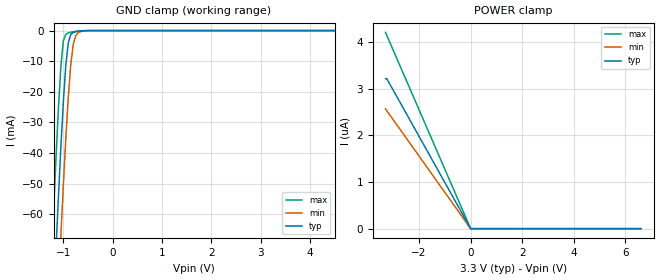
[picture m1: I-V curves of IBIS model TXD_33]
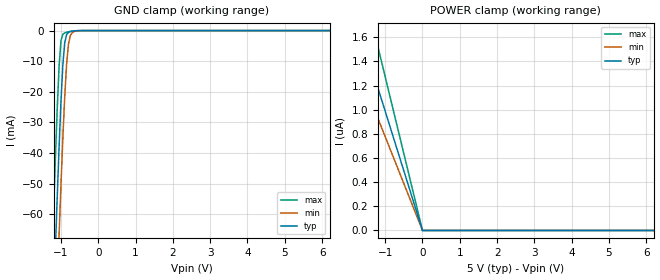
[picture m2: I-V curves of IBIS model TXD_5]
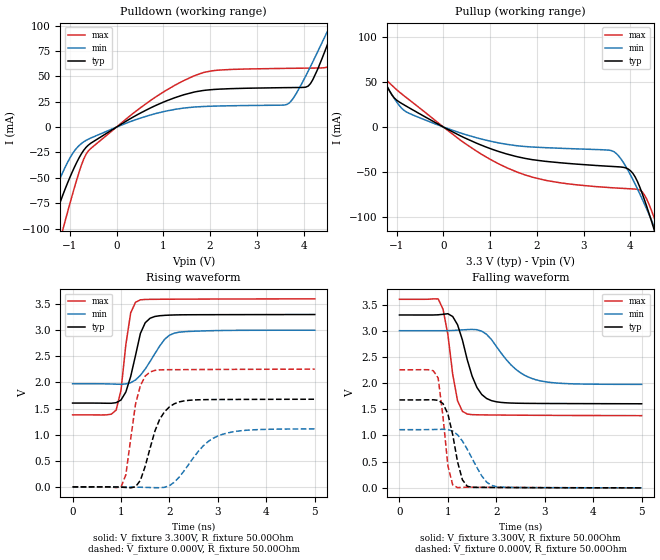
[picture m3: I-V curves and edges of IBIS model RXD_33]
| Texas Instruments Incorporated
| Isolated CAN Transceiver
| Marketing part#   Voltage Range   Package-type   #pins/pkg drawing
| ISO1050DUBR   3V - 5.5V   SOP   8-pin DUB
[IBIS Ver]   4.0
[File name]   iso1050.ibs
[File Rev]   1.0
[Date]   09/04/2009
[Source]   Model built from TISPICED simulations at:
   Texas Instruments Incorporated.
   Analog-eLab, HPA
   12500 TI Blvd
   Dallas, TX -75243
   For Support e-mail: elab_ibis@list.ti.com
[Notes]   Revision History
   Rev 1.0: 09/04/2009
   - Initial model not matched to silicon
   - ccomp values are based on PVT settings:
   MIN: Low Voltage, High Temperature, Weak Process
   TYP: Nominal Voltage, Nominal Temperature, Nominal Process
   MAX: High Voltage, Low Temperature, Fast Process
   - User may change ccomp in the order of number values as
   per end simulator used
[Disclaimer] This model is designed as an aid for customers of Texas Instruments.
 TI and its licensors and suppliers make no warranties, either expressed
 or implied, with respect to this  model, including the warranties of
 merchantability or fitness for a particular purpose.
 The model is provided solely on an "as is" basis. The entire risk as to
 its quality and performance is with the customer.
[Copyright] (C)Copyright 2009 Texas Instruments Incorporated.
   All rights reserved.
|   Component ISO1050
[Component]   ISO1050
[Manufacturer]  Texas Instruments Incorporated
[Package]   |8-pin SOP DUB package
|   typ   min   max
R_pkg   0.115425   0.06126   0.16959
L_pkg   3.423325nH   2.82589nH   4.02076nH
C_pkg   0.799005pF   0.76897pF   0.82904pF
[Pin] signal_name   model_name   R_pin   L_pin   C_pin
   1  VCC1   POWER   0.05706   3.37557nH   0.79052pF
   2  RXD   RXD   0.07605   2.98666nH   0.82904pF
   3  TXD   TXD   0.06126   2.82589nH   0.80903pF
   4  GND1   GND   0.05448   4.63300nH   0.95047pF
   5  GND2   GND   0.04985   5.19150nH   1.01772pF
   6  CANL   CANL_BI   0.16959   4.02076nH   0.76897pF
   7  CANH   CANH_BI   0.06820   2.91438nH   0.81679pF
   8  VCC2   POWER   0.03923   4.28592nH   1.03311pF
[Diff_pin]   inv_pin   vdiff   tdelay_typ   tdelay_min   tdelay_max
| The CANH and CANL are Diff_pins
7   6   0.9V   0 0 0
[Pin Mapping]pulldown_ref pullup_ref gnd_clamp_ref power_clamp_ref |ext_ref
1   NC   PWRBUS1  |VCC1
2   GNDBUS1   PWRBUS1   GNDBUS1   PWRBUS1
3   NC   NC   GNDBUS1   PWRBUS1
4   GNDBUS1   NC   |GND1
5   GNDBUS2   NC   |GND2 to CANH/CANL
6   GNDBUS2   NC   GNDBUS2   PWRBUS2  |CANL has no pullup
7   NC   PWRBUS2   GNDBUS2   PWRBUS2  |CANH has no pulldown
8   NC   PWRBUS2  |VCC2 to CANH/CANL
[Model Selector] TXD
TXD_33   TXD Input model for 3.0V - 3.6V
TXD_5   TXD Input model for 4.5V - 5.5V
[Model Selector] RXD
RXD_33   RXD Output model for 3.0V - 3.6V
RXD_5   RXD Output model for 4.5V - 5.5V
| Models and submodels in the file (6): TXD_33 (Input), TXD_5 (Input), RXD_33 (Output), RXD_5 (Output), CANH_BI (I/O_open_source), CANL_BI (I/O_open_drain)
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|   TXD_33 Model
[Model]   TXD_33
Model_type   Input
|Signals   RXD
Vinh = 2.0
Vinl = 0.8
|   typ   min   max
C_comp   0.6217pF   0.6712pF   0.5756pF
|   typ   min   max
[Voltage Range]   3.3V   3.0V   3.6V
[Temperature Range]   40.0   125.0   -55.0
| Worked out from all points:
|   GND clamp passes 1 mA (typ) near -0.83 V on its own axis
[GND Clamp]
|   Voltage   I(typ)   I(min)   I(max)
-3.3V     -896mA     -941.7mA   -892.3mA
-1.25V    -107.4mA   -137.4mA   -77.4mA
-1.2V     -89.12mA   -119.2mA   -59.18mA
-1.15V    -71.29mA   -101.2mA   -41.62mA
-1.1V     -54.06mA   -83.57mA   -25.26mA
-1.05V    -37.76mA   -66.5mA    -11.46mA
-1V       -23.03mA   -50.19mA   -3.269mA
-950mV    -11.14mA   -35mA      -1.197mA
-900mV    -3.932mA   -21.61mA   -785uA
-800mV    -612.2uA   -4.508mA   -387.7uA
-600mV    -46.68uA   -168.3uA   -47.31uA
6.6V      0A         0A         0A
[POWER Clamp]
|   Voltage   I(typ)   I(min)   I(max)
-3.3V     3.211uA    2.564uA    4.201uA
-3.25V    3.211uA    2.525uA    4.138uA
0V        0A         0A         0A
6.6V      0A         0A         0A
|   TXD_5 Model
[Model]   TXD_5
Model_type   Input
|Signals   TXD
Vinh = 2.0
Vinl = 0.8
|   typ   min   max
C_comp   0.5878pF   0.6309pF   0.5481pF
|   typ   min   max
[Voltage Range]   5.0V   4.5V   5.5V
[Temperature Range]   40.0   125.0   -55.0
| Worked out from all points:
|   GND clamp passes 1 mA (typ) near -0.83 V on its own axis
[GND Clamp]
|   Voltage   I(typ)   I(min)   I(max)
-5V       -1.6A      -1.623A    -1.559A
-1.25V    -107.4mA   -137.4mA   -77.4mA
-1.2V     -89.12mA   -119.2mA   -59.18mA
-1.15V    -71.29mA   -101.2mA   -41.62mA
-1.1V     -54.06mA   -83.57mA   -25.26mA
-1.05V    -37.76mA   -66.5mA    -11.46mA
-1V       -23.04mA   -50.19mA   -3.27mA
-950mV    -11.15mA   -35mA      -1.198mA
-850mV    -1.31mA    -11.07mA   -557.5uA
-750mV    -352.2uA   -1.64mA    -261.2uA
-550mV    -20.4uA    -82.68uA   -21.52uA
10V       0A         0A         0A
[POWER Clamp]
|   Voltage   I(typ)   I(min)   I(max)
-5V       4.941uA    3.885uA    6.302uA
-2.15V    2.125uA    1.671uA    2.737uA
-2.1V     2.075uA    1.632uA    2.674uA
-1.7V     1.68uA     1.321uA    2.164uA
-1.65V    1.63uA     1.282uA    2.101uA
-1.3V     1.285uA    1.01uA     1.655uA
0V        0A         0A         0A
10V       0A         0A         0A
|   RXD_33 MODEL
[Model]   RXD_33
Model_type   Output
| Signals   RXD
Vmeas = 1.55V   |Reference voltage for timing measurements
Cref = 15pF   |Timing specification test load capacitance value
| variable   typ   min   max
|C_comp Average
C_comp   2.5852pF   3.0761pF   2.2483pF
|C_comp Output Low
|C_comp   2.6504pF   3.1260pF   2.3554pF
|C_comp Output High
|C_comp   2.5200pF   3.0261pF   2.1412pF
|   typ   min   max
[Voltage Range]   3.3V   3.0V   3.6V
[Temperature Range]   40.0   125.0   -55.0
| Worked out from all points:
|   slope of the pulldown table from 0 to 0.495 V, typ, clamps not added: 36.9 ohm
|   slope of the pullup table from 0 to 0.495 V, typ, clamps not added: 38.1 ohm
|   falling waveform, V_fixture 3.300V, R_fixture 50.00Ohm: 20-80 % time 334ps typ, 600ps min, 215ps max; typ from 3.3 V to 1.6 V
|   rising waveform, V_fixture 3.300V, R_fixture 50.00Ohm: 20-80 % time 269ps typ, 440ps min, 178ps max; typ from 1.6 V to 3.3 V
|   rising waveform, V_fixture 0.000V, R_fixture 50.00Ohm: 20-80 % time 354ps typ, 601ps min, 230ps max; typ from 0 V to 1.68 V
|   falling waveform, V_fixture 0.000V, R_fixture 50.00Ohm: 20-80 % time 229ps typ, 400ps min, 158ps max; typ from 1.68 V to 0 V
[Pulldown]
|   Voltage   I(typ)   I(min)   I(max)
-3.3V     -444mA     -323.4mA   -559.5mA
-1.65V    -147.4mA   -102.5mA   -196.8mA
-1.35V    -95.7mA    -66.33mA   -136mA
-1.15V    -67.06mA   -44.62mA   -101.2mA
-600mV    -17.67mA   -11.86mA   -23.39mA
1.65V     34.39mA    19.71mA    50.29mA
3.65V     38.89mA    22.42mA    57.89mA
4.15V     42.92mA    59.74mA    58.14mA
4.55V     85.96mA    98.03mA    60.72mA
4.65V     98.18mA    107.5mA    71.46mA
4.85V     122.5mA    126mA      101.8mA
6.6V      280.4mA    243.7mA    322.1mA
[Pullup]
|   Voltage   I(typ)   I(min)   I(max)
-3.3V     239.5mA    206.9mA    282.1mA
-1.95V    129.9mA    113.6mA    151.3mA
-1.7V     102.1mA    91.19mA    115.7mA
-1.3V     55.75mA    53.78mA    58.94mA
-1V       29.98mA    27.94mA    41.63mA
0V        124.8pA    622.4pA    79.46pA
1.35V     -29.93mA   -19.18mA   -45.19mA
3.65V     -44.04mA   -27.51mA   -67.78mA
4.05V     -51.38mA   -58.2mA    -68.97mA
4.3V      -80.92mA   -85.71mA   -75.5mA
4.55V     -121.4mA   -116mA     -107.4mA
6.6V      -493.8mA   -392mA     -570.7mA
[Ramp]
R_load = 50.00Ohm
|   typ   min   max
dV/dt_r   1.007V/353.701ps 666.318mV/600.696ps   1.353V/229.593ps
dV/dt_f   1.017V/334.234ps 614.806mV/599.733ps   1.333V/215.151ps
[Falling Waveform]
V_fixture = 3.300V
V_fixture_min = 3.000V
V_fixture_max = 3.600V
R_fixture = 50.00Ohm
|   Time   V(typ)   V(min)   V(max)
0s        3.3V       3V         3.6V
800ps     3.304V     3V         3.606V
900ps     3.313V     3V         3.41V
1ns       3.324V     3.001V     2.928V
1.2ns     3.113V     3.01V      1.661V
1.4ns     2.445V     3.021V     1.408V
1.6ns     1.915V     3.019V     1.395V
1.9ns     1.665V     2.831V     1.391V
2.8ns     1.612V     2.068V     1.385V
5ns       1.605V     1.975V     1.379V
[Rising Waveform]
V_fixture = 3.300V
V_fixture_min = 3.000V
V_fixture_max = 3.600V
R_fixture = 50.00Ohm
|   Time   V(typ)   V(min)   V(max)
0s        1.605V     1.975V     1.379V
900ps     1.613V     1.967V     1.471V
1ns       1.664V     1.965V     1.851V
1.1ns     1.817V     1.971V     2.723V
1.2ns     2.114V     1.995V     3.333V
1.4ns     2.937V     2.136V     3.582V
1.6ns     3.229V     2.4V       3.591V
1.9ns     3.284V     2.825V     3.593V
2.1ns     3.292V     2.943V     3.594V
5ns       3.3V       3V         3.6V
[Rising Waveform]
V_fixture = 0.000V
V_fixture_min = 0.000V
V_fixture_max = 0.000V
R_fixture = 50.00Ohm
|   Time   V(typ)   V(min)   V(max)
0s        336.7pV    705.2pV    374.2pV
1ns       -5.097mV   157.2uV    -2.804mV
1.1ns     -10.77mV   -533.8uV   231mV
1.3ns     2.172mV    -3.954mV   1.586V
1.4ns     125.6mV    -6.338mV   1.939V
1.6ns     740.1mV    -11.61mV   2.201V
1.8ns     1.298V     -16.07mV   2.24V
2.2ns     1.626V     186mV      2.245V
3ns       1.673V     975.1mV    2.249V
5ns       1.678V     1.111V     2.254V
[Falling Waveform]
V_fixture = 0.000V
V_fixture_min = 0.000V
V_fixture_max = 0.000V
R_fixture = 50.00Ohm
|   Time   V(typ)   V(min)   V(max)
0s        1.678V     1.111V     2.254V
700ps     1.681V     1.113V     2.235V
800ps     1.67V      1.116V     2.097V
1ns       1.412V     1.112V     422.2mV
1.1ns     1.014V     1.084V     56.58mV
1.2ns     495.5mV    1.013V     4.556mV
1.3ns     153.7mV    894mV      9.242mV
1.4ns     30.49mV    736.9mV    12.55mV
1.9ns     7.265mV    47.26mV    9.425mV
5ns       336.7pV    705.2pV    374.2pV
